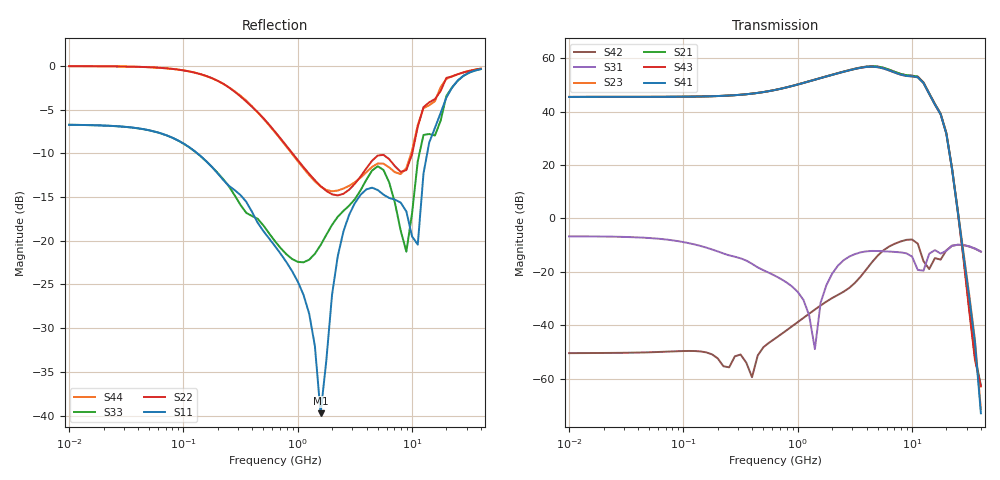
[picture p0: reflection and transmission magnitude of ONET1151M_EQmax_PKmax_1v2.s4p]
! Touchstone Ver. 1.0
! Thu Sep  6 16:11:15 2012
! Number of ports is 4
# Hz	S	DB	R	50.000000
! SCATTERING PARAMETERS  :
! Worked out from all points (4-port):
!   73 points, 10 MHz to 40 GHz, reference 50 ohm
!   strongest paths, dB at 10 MHz, 79.43 MHz, 631 MHz, 5.012 GHz, 40 GHz:
!     S41: 45.4, 45.5, 48.0, 56.6, -72.9
!     S43: 45.4, 45.5, 48.0, 56.6, -62.8
!     S21: 45.5, 45.5, 48.1, 56.8, -62.4
!     S23: 45.5, 45.5, 48.1, 56.8, -71.3
!     S31: -6.7, -8.1, -21.4, -12.2, -12.4
!     S42: -50.4, -49.7, -44.9, -13.9, -12.4
!   lowest |S11| = -39.7 dB at 1.585 GHz (marker M1), VSWR 1.02, Z = 49 - j0.348 ohm
!   |S11| at or under -10 dB: 132.2 MHz to 13.59 GHz (13.46 GHz wide, 196 % of centre)
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1e7  -6.75 -4.6  -110.78 178.1  -6.68 -4.3  -110.74 178.1
     45.46 -175.2  -0.05 7.1  45.46 4.8  -50.53 9.4
     -6.67 -4.3  -110.76 178.0  -6.75 -4.6  -110.76 178.2
     45.44 4.8  -50.35 9.5  45.44 -175.2  -0.05 7.1
1.584893e9  -39.73 -159.9  -40.84 67.0  -22.26 -47.4  -40.77 67.1
            52.55 149.5  -13.75 -84.1  52.54 -30.6  -35.90 47.8
            -31.53 79.5  -40.81 67.1  -20.50 -66.6  -40.78 67.1
            52.49 -31.2  -32.54 36.8  52.48 148.8  -13.80 -81.7
4.466836e9  -13.93 -122.4  -38.30 -11.4  -13.55 53.0  -38.25 -11.1
            56.95 2.6  -10.85 -129.0  56.94 -177.4  -15.25 -135.1
            -12.14 -111.6  -38.28 -11.0  -11.98 64.3  -38.25 -11.4
            56.77 -178.9  -16.33 -142.2  56.75 1.1  -11.56 -132.3
6.309573e9  -15.11 98.5  -37.32 -40.1  -17.68 -67.1  -37.27 -39.6
            55.65 -91.2  -10.67 171.3  55.64 88.9  -9.48 142.0
            -12.37 123.6  -37.31 -39.6  -13.33 -43.4  -37.25 -39.9
            55.37 87.8  -10.47 140.8  55.35 -92.1  -11.62 174.0
7.943282e9  -15.64 23.9  -38.07 -63.6  -20.14 158.4  -38.02 -63.1
            54.07 -163.7  -12.12 136.9  54.05 16.4  -7.96 93.4
            -12.68 63.1  -38.08 -63.0  -18.81 -114.1  -37.97 -63.6
            53.80 15.6  -8.60 94.9  53.78 -164.3  -12.37 142.2
1.122018e10  -20.44 24.8  -40.21 -99.6  -15.18 41.7  -40.25 -98.6
             53.05 41.9  -6.98 85.1  53.04 -137.9  -9.57 10.8
             -19.22 -53.5  -40.30 -97.8  -10.90 58.7  -40.14 -100.2
             52.81 -138.9  -9.42 12.6  52.78 41.3  -6.77 83.0
4e10  -0.38 -143.6  -68.85 138.7  -12.36 -53.0  -68.65 138.6
      -62.42 -171.1  -0.33 -143.9  -71.32 -67.8  -12.41 -53.2
      -12.36 -53.0  -68.57 138.3  -0.38 -143.6  -68.84 139.0
      -72.86 -75.1  -12.41 -53.3  -62.80 -169.8  -0.33 -143.9
